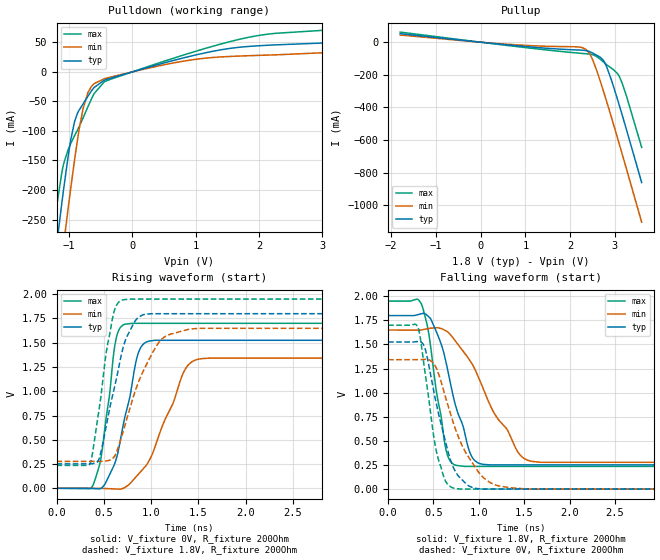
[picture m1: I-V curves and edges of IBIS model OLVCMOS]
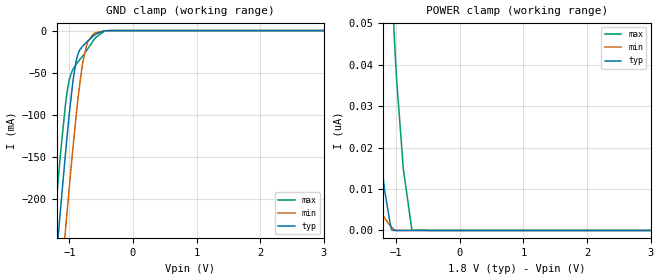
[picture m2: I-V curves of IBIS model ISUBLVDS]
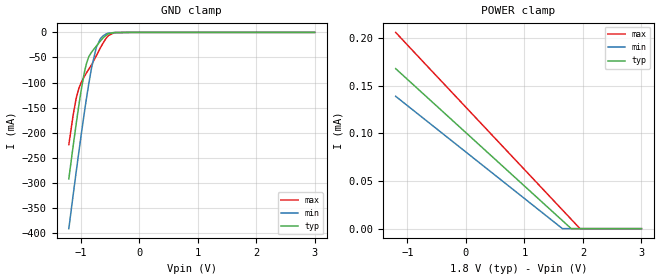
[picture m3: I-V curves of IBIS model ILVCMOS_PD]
|Texas Instruments Incorporated
[IBIS Ver]   4.1
[File name]   p98_sst_dmd.ibs
[File Rev]   1.1
[Date]   01/29/2020
[Source]
| Texas Instruments Incorporated.
| 12500 TI Blvd
| Dallas, TX -75243
[Notes]   Revision History:
| Rev 1.0: 02/28/2019
| - Initial version of the model
| - Model generated from simulations in SPECTRE
| - C_comp although listed in numerical order of value are
|   obtained from varying PVT conditions. For PVT conditions for
|   each specific value refer the buffer description under
|   respective [Model]. IBIS model user is responsible for using
|   appropriate C_comp to simulate for Signal Integrity.
| Rev 1.1: 01/29/2020
| - Removed HSSI interface pins
[Disclaimer]
| This model is designed as an aid for customers of Texas Instruments.
| TI and its licensors and suppliers make no warranties, either expressed
| or implied, with respect to this  model, including the warranties of
| merchantability or fitness for a particular purpose. The model is
| provided solely on an "as is" basis. The entire risk as to its quality
| and performance is with the customer.
| In order to provide better modelling of the HSSI interface,
| these pins have been removed from this IBIS model.  It is recommended
| that the package s-parameters and HSSI input hspice models are used
| to model the HSSI interface.
| This model simulates to CMOS voltage and temperature limits that are beyond the
| limits of the DMD. There is no implication that the DMD can be run to these limits.
| This model is subject to change without notice. Texas Instruments
| Incorporated is not responsible for updating this model.
[Copyright]
 (C) Copyright 2020 Texas Instruments Incorporated. All rights reserved.
|   Device
[Component] P98_SST_DMD
[Manufacturer]   TI
[Package]
| variable   typ   min   max
R_pkg   0.05   0.04   0.06
L_pkg   1.0nH   0.8nH   1.2nH
C_pkg   0.2pF   0.16pF   0.24pF
[Pin]  signal_name   model_name   R_pin   L_pin   C_pin
A27   LS_WDATA_N   ISUBLVDS   NA   NA   NA
B26   LS_WDATA_P   ISUBLVDS   NA   NA   NA
A25   LS_CLK_N   ISUBLVDS   NA   NA   NA
B24   LS_CLK_P   ISUBLVDS   NA   NA   NA
AE23   DMD_DEN_ARSTZ   term   NA   NA   NA
E27   DMD_DEN_ARSTZ   ILVCMOS_PD   NA   NA   NA
Y4   DMD_DEN_ARSTZ   term   NA   NA   NA
F24   LS_RDATA_A   OLVCMOS   NA   NA   NA
D26   LS_RDATA_B   OLVCMOS   NA   NA   NA
F30   LS_RDATA_C   OLVCMOS   NA   NA   NA
C27   LS_RDATA_D   OLVCMOS   NA   NA   NA
E29   DMUX_OUT   OLVCMOS   NA   NA   NA
[Diff Pin]  inv_pin  vdiff  tdelay_typ tdelay_min tdelay_max
B26   A27   100mV   NA   NA   NA
B24   A25   100mV   NA   NA   NA
|Differential termination for SUBLVDS inputs and internally connecting DMD_DEN_ARSTZ pins
[Series Pin Mapping] pin_2 model_name
B26   A27   SeriesR
B24   A25   SeriesR
AE23  E27   SeriesR_conn
Y4   E27   SeriesR_conn
[Model] SeriesR
Model_type Series
C_comp   0   0   0
[Voltage Range]  1.80  1.65  1.95
[Temperature Range] 25   125   -55
[R Series]   100   80   110
[Model] SeriesR_conn
Model_type Series
C_comp   0   0   0
[Voltage Range]  1.80  1.65  1.95
[Temperature Range] 25   125   -55
[R Series]   2   1.5   2.5
[Model]  term
Model_type Terminator
C_comp   0   0   0
[Voltage Range]  3.30  3.00  3.60
[Temperature Range] 25   85   -40
| Models and submodels in the file (6): SeriesR (Series), SeriesR_conn (Series), OLVCMOS (Output), ISUBLVDS (Input), ILVCMOS_PD (Input), term (Terminator)
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|   Model
[Model]   OLVCMOS
Model_type   Output
Polarity   Non-Inverting
Vmeas = 0.9
Vref = 0
Cref = 2pF
Rref = 1000000
|   typ   min   max
C_comp   1.57686pF   1.41042pF   1.72855pF
[Voltage Range]   1.8   1.65   1.95
[Temperature Range]   25   125   -55
[Pullup Reference]   1.8   1.65   1.95
[Pulldown Reference]   0   0   0
[Power Clamp Reference]   1.8   1.65   1.95
[GND Clamp Reference]   0   0   0
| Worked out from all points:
|   slope of the pulldown table from 0 to 0.27 V, typ, clamps not added: 32.5 ohm
|   slope of the pullup table from 0 to 0.27 V, typ, clamps not added: 35.9 ohm
|   falling waveform, V_fixture 1.8V, R_fixture 200Ohm: 20-80 % time 260ps typ, 475ps min, 159ps max; typ from 1.8 V to 0.251 V
|   rising waveform, V_fixture 0V, R_fixture 200Ohm: 20-80 % time 191ps typ, 328ps min, 126ps max; typ from 0 V to 1.53 V
|   rising waveform, V_fixture 1.8V, R_fixture 200Ohm: 20-80 % time 206ps typ, 310ps min, 152ps max; typ from 0.251 V to 1.8 V
|   falling waveform, V_fixture 0V, R_fixture 200Ohm: 20-80 % time 225ps typ, 336ps min, 160ps max; typ from 1.53 V to 0 V
[Pulldown]
|   Voltage   I(typ)   I(min)   I(max)
-1.8V     -860.9mA   -959.8mA   -788.9mA
-1.238V   -329.6mA   -428.5mA   -262mA
-1.184V   -281.3mA   -379.2mA   -217.9mA
-1.087V   -198.1mA   -292.3mA   -155.5mA
-1.017V   -143.5mA   -231.7mA   -131.7mA
-914.4mV  -84.12mA   -148.6mA   -107.9mA
-779.4mV  -54.23mA   -61.75mA   -77.9mA
-606.6mV  -26.47mA   -20.12mA   -36.9mA
-401.4mV  -12.54mA   -10.32mA   -14.75mA
1.597V    40.48mA    26.35mA    52.67mA
3.055V    49mA       32.57mA    70.62mA
3.6V      52.73mA    48.36mA    73.02mA
[Pullup]
|   Voltage   I(typ)   I(min)   I(max)
-1.8V     52.3mA     44.12mA    62.11mA
689.4mV   -18.71mA   -14.27mA   -23.08mA
2.164V    -47.69mA   -28.71mA   -66.39mA
2.358V    -51.6mA    -44.58mA   -70.93mA
2.434V    -57.52mA   -69.05mA   -72.93mA
2.509V    -67.22mA   -111.6mA   -76.97mA
2.747V    -112.3mA   -301.8mA   -121.6mA
2.822V    -154.6mA   -369.1mA   -139.3mA
2.92V     -229mA     -457.8mA   -158.8mA
3.092V    -380.8mA   -618.9mA   -206.4mA
3.254V    -531.3mA   -772.5mA   -325.1mA
3.6V      -861.7mA   -1.105A    -645.8mA
[Ramp]
R_load = 200
|   typ   min   max
dV/dt_r   0.915753/1.90736e-10   0.805642/3.27008e-10   1.01994/1.26276e-10
dV/dt_f   0.929328/2.59765e-10   0.824077/4.7559e-10   1.02849/1.58948e-10
[Falling Waveform]
V_fixture = 1.8V
V_fixture_min = 1.65V
V_fixture_max = 1.95V
R_fixture = 200Ohm
C_fixture = 0F
|   Time   V(typ)   V(min)   V(max)
0s        1.8V       1.65V      1.95V
365.5ps   1.818V     1.651V     1.924V
449.3ps   1.786V     1.666V     1.607V
641.5ps   1.302V     1.639V     395mV
843.3ps   588.6mV    1.41V      236.1mV
912.6ps   354.8mV    1.318V     236.1mV
1.012ns   264.5mV    1.125V     236.1mV
1.435ns   251.8mV    378.3mV    236.1mV
1.683ns   251.8mV    278.6mV    236.1mV
50ns      251.1mV    276.5mV    235.9mV
[Rising Waveform]
V_fixture = 0V
V_fixture_min = 0V
V_fixture_max = 0V
R_fixture = 200Ohm
C_fixture = 0F
|   Time   V(typ)   V(min)   V(max)
0s        -19.49nV   1.791nV    -147.3nV
386.3ps   -3.017mV   -193.2uV   31.51mV
472.3ps   120.4uV    -633.8uV   322.1mV
631.9ps   301.8mV    -7.552mV   1.548V
804.3ps   1.105V     77.06mV    1.7V
869.3ps   1.405V     148.2mV    1.7V
955ps     1.51V      244.8mV    1.7V
1.366ns   1.525V     1.233V     1.7V
1.629ns   1.525V     1.342V     1.7V
50ns      1.526V     1.343V     1.7V
[Rising Waveform]
V_fixture = 1.8V
V_fixture_min = 1.65V
V_fixture_max = 1.95V
R_fixture = 200Ohm
C_fixture = 0F
|   Time   V(typ)   V(min)   V(max)
0s        251.1mV    276.5mV    235.9mV
358.6ps   251.9mV    277.1mV    261.4mV
452.2ps   310.3mV    277.2mV    826.9mV
525.3ps   637.3mV    282.3mV    1.395V
602.1ps   993.9mV    315.2mV    1.795V
772.9ps   1.617V     810.8mV    1.95V
869.3ps   1.765V     1.099V     1.95V
1.103ns   1.799V     1.527V     1.95V
1.535ns   1.799V     1.649V     1.95V
50ns      1.8V       1.65V      1.95V
[Falling Waveform]
|Gnd
V_fixture = 0V
V_fixture_min = 0V
V_fixture_max = 0V
R_fixture = 200Ohm
C_fixture = 0F
|   Time   V(typ)   V(min)   V(max)
0s        1.526V     1.343V     1.7V
324.9ps   1.531V     1.343V     1.686V
409.1ps   1.453V     1.347V     1.196V
503.2ps   1.018V     1.302V     544.1mV
547.3ps   817.9mV    1.218V     332.3mV
654.5ps   412.1mV    885.3mV    51.44mV
804.3ps   108.2mV    475.6mV    1.209mV
1.092ns   1.644mV    87.59mV    1.202mV
1.535ns   1.629mV    1.877mV    1.191mV
50ns      -19.49nV   1.791nV    -107.8nV
|   Model
[Model]   ISUBLVDS
Model_type   Input
Vinl = 0.54
Vinh = 1.26
|   typ   min   max
C_comp   1.17267pF   1.10975pF   1.26901pF
[Voltage Range]   1.8   1.65   1.95
[Temperature Range]   25   125   -55
[Power Clamp Reference]   1.8   1.65   1.95
[GND Clamp Reference]   0   0   0
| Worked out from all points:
|   GND clamp passes 1 mA (typ) near -0.47 V on its own axis
[GND Clamp]
|   Voltage   I(typ)   I(min)   I(max)
-1.8V     -836mA     -928.2mA   -769mA
-1.26V    -322.6mA   -416.8mA   -253.8mA
-1.222V   -288.1mA   -382.2mA   -219.7mA
-1.179V   -249.1mA   -342.9mA   -181.6mA
-1.06V    -146.6mA   -237.5mA   -88.17mA
-995.4mV  -95.98mA   -182.4mA   -56.72mA
-892.8mV  -36.76mA   -101.9mA   -40.31mA
-784.8mV  -18.01mA   -36.33mA   -29.87mA
-714.6mV  -12.92mA   -14.02mA   -22.27mA
-617.4mV  -6.056mA   -3.892mA   -11.4mA
-369mV    -45.26uA   -40.26uA   -81.57uA
3.6V      0A         0A         0A
[POWER Clamp]
|   Voltage   I(typ)   I(min)   I(max)
-1.8V     372.1nA    94.94nA    1.561uA
-1.676V   214.4nA    48.37nA    997.5nA
-1.546V   117.4nA    26.07nA    607.7nA
-1.4V     53.84nA    12.25nA    330.4nA
-1.373V   45.77nA    10.55nA    293nA
-1.233V   16.53nA    4.419nA    150.3nA
-1.071V   160.3pA    802pA      61.15nA
-1.033V   0A         252.1pA    48.05nA
-995.4mV  0A         0A         37.08nA
-887.4mV  0A         0A         14.92nA
-752.4mV  0A         0A         139.4pA
3.6V      0A         0A         0A
|   Model
[Model]   ILVCMOS_PD
Model_type   Input
Vinl = 0.54
Vinh = 1.26
|   typ   min   max
C_comp   1.48655pF   1.46519pF   1.50106pF
[Voltage Range]   1.8   1.65   1.95
[Temperature Range]   25   125   -55
[Power Clamp Reference]   1.8   1.65   1.95
[GND Clamp Reference]   0   0   0
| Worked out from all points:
|   GND clamp passes 1 mA (typ) near -0.45 V on its own axis
[GND Clamp]
|   Voltage   I(typ)   I(min)   I(max)
-1.2V     -292.2mA   -391.6mA   -224mA
-1.124V   -225.3mA   -323.1mA   -164.1mA
-1.066V   -175.4mA   -270.9mA   -127.4mA
-985.8mV  -113.4mA   -202.2mA   -99.54mA
-901.8mV  -63.66mA   -134.3mA   -81.49mA
-809.4mV  -39.13mA   -69.61mA   -64.06mA
-733.8mV  -28.06mA   -31.81mA   -47.47mA
-662.4mV  -17.41mA   -13.01mA   -31.28mA
-612mV    -10.76mA   -6.62mA    -20.69mA
-519.6mV  -2.756mA   -1.491mA   -6.014mA
-423mV    -305.6uA   -206.9uA   -613.5uA
3V        0A         0A         0A
[POWER Clamp]
|   Voltage   I(typ)   I(min)   I(max)
-1.2V     167.8uA    138.8uA    205.8uA
1.648V    8.514uA    108.4nA    19.73uA
1.799V    58.82nA    0A         9.863uA
1.946V    0A         0A         265.9nA
3V        0A         0A         0A
